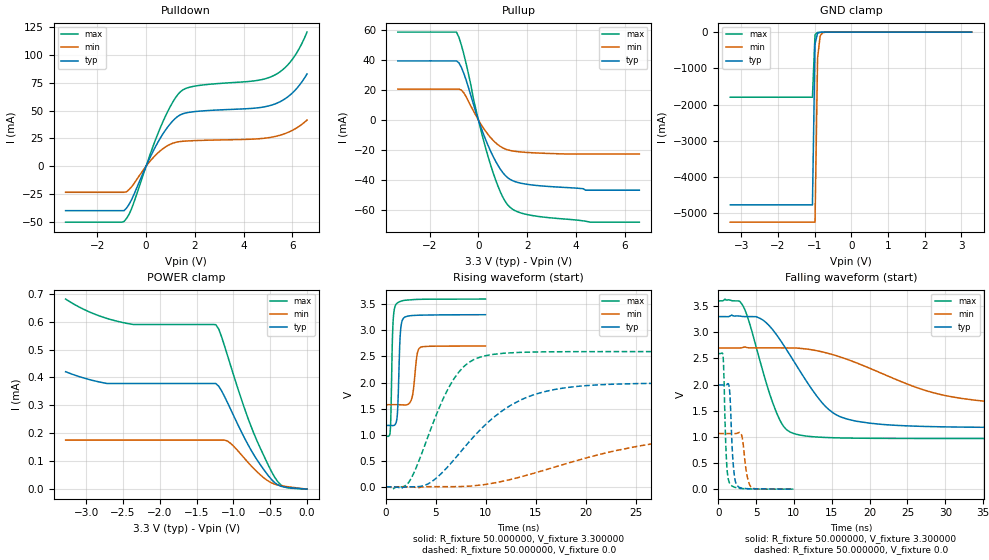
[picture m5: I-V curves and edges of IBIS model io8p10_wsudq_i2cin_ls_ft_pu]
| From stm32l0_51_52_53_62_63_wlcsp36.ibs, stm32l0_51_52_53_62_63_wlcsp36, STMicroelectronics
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|   Model io8p10_wsudq_i2cin_ls_ft_pu
[Model]  io8p10_wsudq_i2cin_ls_ft_pu
Model_type I/O
Polarity   Non-Inverting
Enable   Active-Low
Vinl =   0.990000V
Vinh =   2.310000V
Vmeas =  1.650000V
Cref =   50.000000pF
Rref =   100.000000M
Vref =   0.0V
C_comp   3.020400pF   2.988300pF   3.054500pF
[Temperature Range]   25.000000   0.125000k   -40.000000
[Pullup Reference]   3.300000V   2.700000V   3.600000V
[Pulldown Reference]   0.0V   0.0V   0.0V
[POWER Clamp Reference]   3.300000V   2.700000V   3.600000V
[GND Clamp Reference]   0.0V   0.0V   0.0V
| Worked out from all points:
|   slope of the pulldown table from 0 to 0.495 V, typ, clamps not added: 22.6 ohm
|   slope of the pullup table from 0 to 0.495 V, typ, clamps not added: 23.9 ohm
|   GND clamp passes 1 mA (typ) near -0.64 V on its own axis
|   rising waveform, R_fixture 50.000000, V_fixture 3.300000: 20-80 % time 221ps typ, 368ps min, 182ps max; typ from 1.18 V to 3.3 V
|   rising waveform, R_fixture 50.000000, V_fixture 0.0: 20-80 % time 6.53ns typ, 13.7ns min, 3.48ns max; typ from 0.001 V to 1.99 V
|   falling waveform, R_fixture 50.000000, V_fixture 3.300000: 20-80 % time 5.96ns typ, 12.5ns min, 3.28ns max; typ from 3.3 V to 1.18 V
|   falling waveform, R_fixture 50.000000, V_fixture 0.0: 20-80 % time 411ps typ, 575ps min, 334ps max; typ from 1.99 V to 0.001 V
[Pulldown]
|Voltage   I(typ)   I(min)   I(max)
-3.3V     -39.83mA   -23.37mA   -50.2mA
-900mV    -39.83mA   -23.37mA   -49.52mA
-600mV    -30.28mA   -18.59mA   -38.45mA
100mV     4.867mA    2.821mA    6.48mA
600mV     25.85mA    14.17mA    35.39mA
1V        38.33mA    19.81mA    53.88mA
1.4V      46.1mA     22.18mA    66.72mA
2V        49.07mA    23.02mA    71.93mA
4.4V      52.05mA    24.38mA    76.53mA
5.2V      55.25mA    26.31mA    81.02mA
6V        65.78mA    32.24mA    95.96mA
6.6V      82.83mA    41.41mA    120.4mA
[Pullup]
|Voltage   I(typ)   I(min)   I(max)
-3.3V     39.53mA    20.64mA    58.82mA
-900mV    39.53mA    20.64mA    58.82mA
-800mV    38.25mA    20.64mA    55.32mA
-600mV    31.26mA    18.2mA     44.19mA
0V        90fA       26pA       0A
500mV     -20.88mA   -11.78mA   -30.07mA
900mV     -32.92mA   -17.72mA   -48.14mA
1.3V      -39.75mA   -20.41mA   -58.47mA
1.8V      -42.5mA    -21.48mA   -62.49mA
2.7V      -44.27mA   -22.29mA   -65.04mA
4.6V      -47mA      -22.8mA    -68.4mA
6.6V      -47mA      -22.8mA    -68.4mA
[GND_clamp]
|Voltage   I(typ)   I(min)   I(max)
-3.3V     -4.766A    -5.244A    -1.797A
-1.06V    -4.766A    -5.244A    -1.797A
-990mV    -326.6mA   -5.244A    -67.9mA
-920mV    -28.92mA   -722.1mA   -10.96mA
-850mV    -6.612mA   -104.2mA   -6.532mA
-780mV    -3.464mA   -17.27mA   -4.209mA
-500mV    -57.88uA   -167.8uA   -34.02uA
3.28V     0A         0A         0A
[POWER_clamp]
|Voltage   I(typ)   I(min)   I(max)
-3.28V    420.5uA    175.8uA    680.6uA
-2.72V    378.4uA    175.8uA    611.4uA
-2.4V     378.3uA    175.8uA    591.2uA
-1.24V    378.3uA    175.8uA    588.9uA
-1.2V     368.9uA    175.8uA    573.6uA
-1.08V    309.6uA    172.2uA    478.3uA
-920mV    220.5uA    131.5uA    344.5uA
-760mV    139.7uA    83.77uA    224.7uA
-480mV    33.95uA    22.2uA     61.82uA
-400mV    15.86uA    14.74uA    27.74uA
-320mV    8.147uA    10.83uA    9.34uA
0V        0A         0A         0A
[Ramp]
| variable   typ   min   max
dV/dt_r  1.19492/6.52763n   0.62981/13.59664n   1.55547/3.47253n
dV/dt_f  1.27302/5.95822n   0.65238/12.42652n   1.57816/3.27370n
R_load = 50.000000
[Rising Waveform]
R_fixture= 50.000000
V_fixture= 3.300000
V_fixture_min= 2.700000
V_fixture_max= 3.600000
|time   V(typ)   V(min)   V(max)
0s        1.178V     1.575V     969.7mV
440.4ps   1.177V     1.575V     1.075V
700.7ps   1.174V     1.575V     3.077V
1.021ns   1.231V     1.576V     3.499V
1.181ns   1.489V     1.576V     3.529V
1.461ns   2.97V      1.574V     3.556V
1.782ns   3.236V     1.57V      3.573V
2.603ns   3.284V     1.699V     3.588V
3.443ns   3.291V     2.671V     3.595V
9.97ns    3.3V       2.7V       3.6V
[Rising Waveform]
R_fixture= 50.000000
V_fixture= 0.0
V_fixture_min= 0.0
V_fixture_max= 0.0
|time   V(typ)   V(min)   V(max)
0s        1.062mV    1.811mV    1.013mV
2.302ns   1.414mV    206.4uV    89.6mV
4.204ns   54.74mV    3.53mV     956.7mV
6.507ns   451.4mV    3.889mV    1.975V
8.008ns   789.7mV    10mV       2.339V
9.71ns    1.144V     39.84mV    2.502V
13.51ns   1.667V     191.4mV    2.578V
18.82ns   1.919V     487.8mV    2.592V
30.93ns   1.99V      928.3mV    2.593V
49.85ns   1.993V     1.064V     2.593V
[Falling Waveform]
R_fixture= 50.000000
V_fixture= 3.300000
V_fixture_min= 2.700000
V_fixture_max= 3.600000
|time   V(typ)   V(min)   V(max)
0s        3.3V       2.7V       3.6V
3.303ns   3.302V     2.711V     3.499V
5.606ns   3.26V      2.702V     2.408V
7.508ns   2.991V     2.702V     1.536V
8.609ns   2.761V     2.701V     1.207V
9.91ns    2.465V     2.701V     1.068V
14.31ns   1.562V     2.605V     988.5mV
18.22ns   1.301V     2.419V     975.9mV
31.13ns   1.19V      1.76V      970mV
49.85ns   1.178V     1.575V     969.7mV
[Falling Waveform]
R_fixture= 50.000000
V_fixture= 0.0
V_fixture_min= 0.0
V_fixture_max= 0.0
|time   V(typ)   V(min)   V(max)
0s        1.993V     1.064V     2.593V
640.6ps   1.993V     1.064V     2.541V
1.101ns   1.998V     1.064V     533.3mV
1.542ns   1.816V     1.064V     105.2mV
1.982ns   485.4mV    1.064V     49.86mV
2.482ns   73.53mV    1.069V     24.51mV
3.143ns   21.14mV    1.005V     12.02mV
3.744ns   11.29mV    313.4mV    9.486mV
4.384ns   7.806mV    34.92mV    5.402mV
9.97ns    1.062mV    1.811mV    1.013mV
